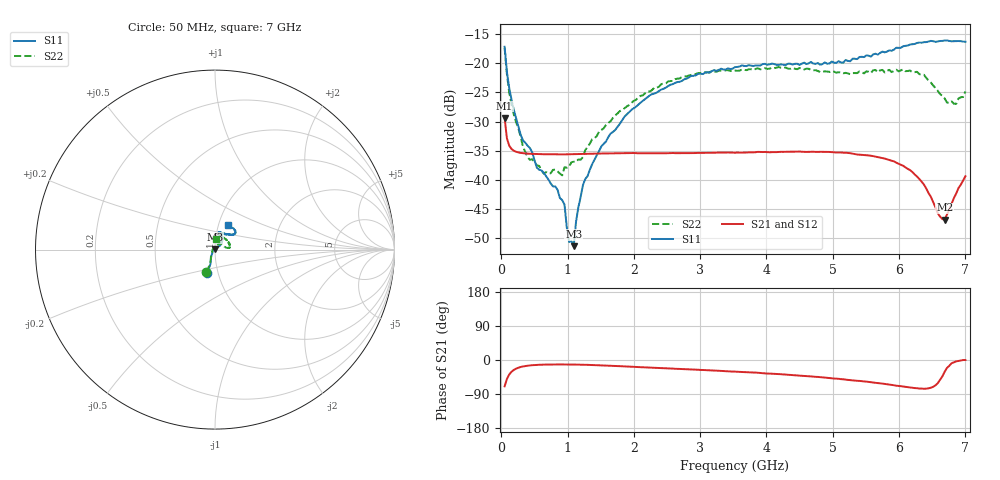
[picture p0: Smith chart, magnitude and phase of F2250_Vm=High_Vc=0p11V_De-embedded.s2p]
! Integrated Device Technology
! Corporate Headquarters
! 6024 Silver Creek Valley Road
! San Jose, CA 95138  USA
! Phone:  1-408-284-8200
! Toll Free:  1-800-223-1366
! Webpage:  http://www.idt.com/
! Timing and RF Division
! 515 Groton Road, Suite 102
! Westford, MA 01886-6024
! Device:  F2250
! Description: Voltage Variable RF Attenuator
! Frequency:  50.0 -  6000.00 MHz
! Package:  3x3 mm Thin QFN Plastic Package: 16 pin
! Ports:  2 RF, 3 DC
!  Pin  1  = GND
!  Pin  2  = NC
!  Pin  3  = RF1  = Port 1
!  Pin  4  = NC
!  Pin  5  = GND
!  Pin  6  = GND
!  Pin  7  = GND
!  Pin  8  = GND
!  Pin  9  = NC
!  Pin 10  = RF2  = Port 2
!  Pin 11  = NC
!  Pin 12  = GND
!  Pin 13  = GND
!  Pin 14  = VCNTRL
!  Pin 15  = VDD
!  Pin 16  = VMODE
! Vcntrl:  0.110 Volts
! Vmode:  +3.300 Volts
! Vdd:  +3.30  Volts
! Current:  1.244 mA
! Data:  The device was measured on a the F2250 evaluation board which has
!  individual transmission lines to the RF pins.  Data was collected
!  using a calibrated network analyzer.  The evaluation board was
!  de-embedded using a TRL calibration technique.
!  The reference plane is the edge of the package pin.
! Misc:  SN 10
!  Action Tracker AT0258
! Date Measured:  2014-11-26
! Date:  2015-10-15  MJV
! Note:
!  Integrated Device Technology supplies this data as a sample of measured
!  data at the package pin for this product.  Your particular data for this
!  product may vary.
!  Data was taken at 25 degrees C.
!  Integrated Device Technology reserves the right to change this data at anytime.
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# GHz S dB R 50
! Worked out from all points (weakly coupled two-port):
!   201 points, 50 MHz to 7 GHz, reference 50 ohm
!   highest |S21| = -29.38 dB at 50 MHz (marker M1); lowest = -46.8 dB at 6.687 GHz (marker M2)
!   lowest |S11| = -51.3 dB at 1.093 GHz (marker M3), VSWR 1.01, Z = 50 + j0.272 ohm
!   |S11| at or under -10 dB: start of sweep to end of sweep
!   |S22| runs from -39.2 to -17.4 dB; largest |S21 - S12| = 5.5e-05
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0.05  -17.18 -108.5  -29.38 -69.5  -29.38 -69.5  -17.37 -110.6
0.08475  -21.47 -107.4  -32.86 -50.1  -32.86 -50.1  -21.87 -109.0
0.15425  -26.23 -116.6  -34.68 -31.0  -34.68 -31.0  -27.11 -120.7
0.29325  -32.28 -127.5  -35.35 -18.4  -35.35 -18.5  -32.66 -133.5
0.3975  -34.13 -142.2  -35.48 -15.1  -35.48 -15.0  -36.09 -158.4
0.5365  -37.88 -154.6  -35.55 -12.9  -35.55 -12.9  -37.48 179.9
0.64075  -38.78 -162.6  -35.58 -12.2  -35.58 -12.2  -38.89 160.6
0.91875  -43.43 155.8  -35.60 -11.8  -35.60 -11.8  -39.19 127.9
0.9535  -44.20 171.0  -35.60 -11.8  -35.60 -11.8  -37.81 124.3
1.023  -50.62 140.2  -35.59 -11.9  -35.59 -11.9  -37.70 107.9
1.0925  -51.32 89.2  -35.57 -12.0  -35.58 -12.0  -36.86 98.8
1.12725  -47.14 61.5  -35.56 -12.1  -35.56 -12.2  -36.90 91.6
1.2315  -40.85 40.8  -35.52 -12.5  -35.53 -12.5  -36.06 77.2
1.6485  -32.03 41.3  -35.44 -15.2  -35.44 -15.2  -29.92 60.1
2.37825  -24.75 46.7  -35.39 -21.0  -35.40 -21.1  -24.02 53.9
3.525  -20.66 71.7  -35.32 -30.6  -35.32 -30.6  -21.26 72.9
4.7065  -20.06 72.0  -35.15 -43.9  -35.16 -43.9  -21.21 70.4
5.85325  -17.79 40.5  -36.58 -64.8  -36.58 -65.0  -21.13 23.3
6.27025  -16.53 39.4  -39.39 -74.5  -39.40 -74.5  -21.46 8.6
6.68725  -16.11 47.9  -46.79 -31.1  -46.77 -30.7  -26.03 28.4
6.861  -16.22 54.5  -42.31 -3.6  -42.27 -3.8  -26.96 57.4
7  -16.32 62.4  -39.35 -0.1  -39.33 -0.3  -24.82 83.6
